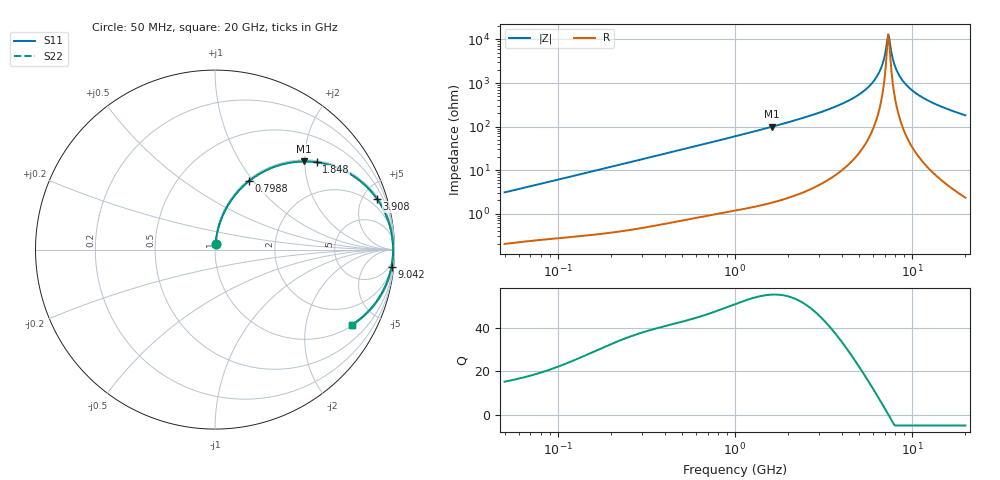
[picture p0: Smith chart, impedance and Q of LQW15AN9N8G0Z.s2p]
!Murata Part Number: LQW15AN9N8G0Z
!These Parameters are Measured in Series Mode Connection
!  o--[Z]--o
!Port1  Port2
!  o-------o
!Freq. Start=50[MHz] Stop=20[GHz], 401[Steps]
# Hz S RI R 50
!Freq.(Hz) S11(Real) S11(Imag) S21(Real) S21(Imag) S12(Real) S12(Imag) S22(Real) S22(Imag)
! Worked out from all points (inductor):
!   401 points, 50 MHz to 20 GHz, reference 50 ohm
!   read as one part in series: L = 9.66 nH near 51.52 MHz
!   highest Q = 55.5 at 1.615 GHz (marker M1), where L = 9.73 nH
!   self-resonance near 7.331 GHz
!   S11 on the Smith chart (normalised r, x): 50 MHz: 1.00, +0.06; 798.8 MHz: 1.02, +0.95; 1.848 GHz: 1.04, +2.29; 3.908 GHz: 1.18, +6.32; 9.042 GHz: 3, -20; 20 GHz: 1.05, -3.62
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5e7  0.00293 0.0304  0.9971 -0.0304  0.9971 -0.0304  0.00293 0.0304
1.364002e8  0.00959 0.0805  0.9904 -0.0805  0.9904 -0.0805  0.00959 0.0805
3.721004e8  0.051 0.2079  0.949 -0.2079  0.949 -0.2079  0.051 0.2079
7.987718e8  0.1878 0.3803  0.8122 -0.3803  0.8122 -0.3803  0.1878 0.3803
1e9  0.2653 0.4318  0.7347 -0.4318  0.7347 -0.4318  0.2653 0.4318
1.614971e9  0.4937 0.491  0.5063 -0.491  0.5063 -0.491  0.4937 0.491
1.848039e9  0.5669 0.4865  0.4331 -0.4865  0.4331 -0.4865  0.5669 0.4865
2.728004e9  0.7669 0.4127  0.2331 -0.4127  0.2331 -0.4127  0.7669 0.4127
3.908127e9  0.9024 0.2827  0.0976 -0.2827  0.0976 -0.2827  0.9024 0.2827
5.041459e9  0.9609 0.1724  0.0391 -0.1724  0.0391 -0.1724  0.9609 0.1724
6.034176e9  0.9838 0.0908  0.0162 -0.0908  0.0162 -0.0908  0.9838 0.0908
6.601595e9  0.9899 0.0495  0.0101 -0.0495  0.0101 -0.0495  0.9899 0.0495
6.905011e9  0.9916 0.0288  0.00844 -0.0288  0.00844 -0.0288  0.9916 0.0288
7.222371e9  0.9924 0.00801  0.00762 -0.00801  0.00762 -0.00801  0.9924 0.00801
7.442007e9  0.9925 -0.00583  0.00755 0.00583  0.00755 0.00583  0.9925 -0.00583
7.554318e9  0.9923 -0.0128  0.00766 0.0128  0.00766 0.0128  0.9923 -0.0128
7.901521e9  0.9914 -0.0335  0.00858 0.0335  0.00858 0.0335  0.9914 -0.0335
8.141811e9  0.9903 -0.0473  0.00969 0.0473  0.00969 0.0473  0.9903 -0.0473
9.041845e9  0.9834 -0.0956  0.0166 0.0956  0.0166 0.0956  0.9834 -0.0956
1.034674e10  0.9672 -0.1571  0.0328 0.1571  0.0328 0.1571  0.9672 -0.1571
1.220001e10  0.936 -0.2306  0.064 0.2306  0.064 0.2306  0.936 -0.2306
2e10  0.7635 -0.4186  0.2365 0.4186  0.2365 0.4186  0.7635 -0.4186
